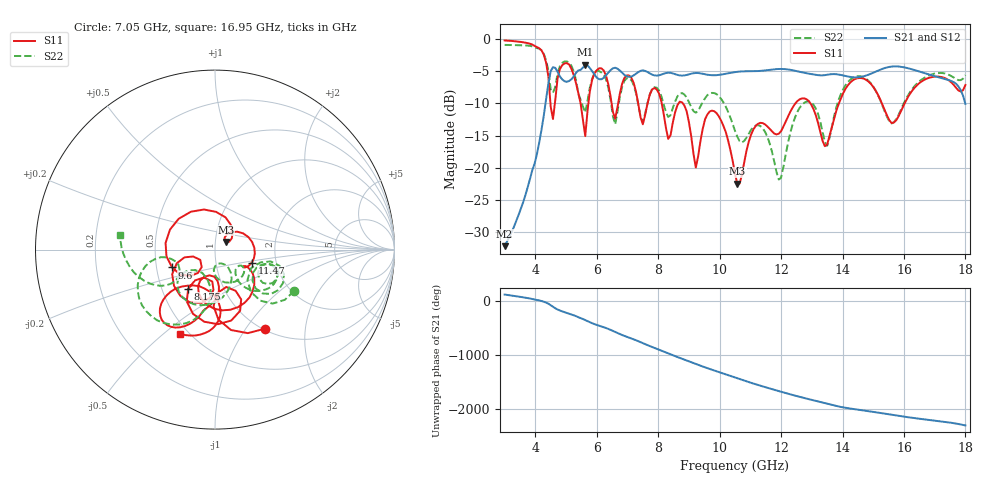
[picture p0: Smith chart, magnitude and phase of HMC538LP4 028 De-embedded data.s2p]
! Chelmsford, MA 01824
! http://www.hittite.com
! Tel: 978-250-3343
! Fax: 978-250-3373
! Device  :  HMC538LP4
! Description:  600 Analog Phase Shifter
! Frequency  :  6.0 GHz - 15.0 GHz
! Package  :  LP4  - 4x4 mm Quad Flatpack No-Lead (QFN) Plastic Package: 24 pin
! Ports  :  2 RF, 1 DC
!  Pin  3  = Rfin  = Port 1
!  Pin  16  = Rfout = Port 2
!  pin  21  = vCTL
! Voltages:  VCTL  = 0 to 5.0 Volts
! Currents :  Vb(V)  Vd(V)  Ib(mA)  Id(mA)
!  0.00  2.80  0.000000	0.471374
! Data:  The device was measured on evaluation board 111296-1.
!  Data was collected using a calibrated network analyzer.
!  The evaluation circuit board was modeled and simulated.This was use
!  to removed the evaluation board circuit from the measured data.
!  The reference plane is the center of the package pin.
! Misc:  Lot #
!Date Measured:  03 - 11 -2009
! Date:  03 - 17 -2009
! Note:
!  Hittite Microwave supplies this data as a sample of measured data at the
!  package pin for this package product.  Your particular data for this product
!  may vary.
!  Data was taken at 25 degrees C.
!  Hittite Microwave reserves the right to change this data at anytime.
# MHz S MA R 50
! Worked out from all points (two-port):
!   201 points, 3 GHz to 18 GHz, reference 50 ohm
!   highest |S21| = -4.00 dB at 5.625 GHz (marker M1); lowest = -32.2 dB at 3 GHz (marker M2)
!   |S21| within 3 dB of the highest: 4.422 GHz to 17.71 GHz (13.28 GHz wide, 120 % of centre)
!   lowest |S11| = -22.5 dB at 10.57 GHz (marker M3), VSWR 1.16, Z = 56.3 + j4.89 ohm
!   |S11| at or under -10 dB: 8.8 GHz to 12.47 GHz (3.668 GHz wide, 34.5 % of centre); 12.95 GHz to 13.88 GHz (929 MHz wide, 6.92 % of centre); 15.28 GHz to 16.02 GHz (743.1 MHz wide, 4.75 % of centre)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
!   |S22| runs from -21.8 to -0.9 dB; largest |S21 - S12| = 0.0022
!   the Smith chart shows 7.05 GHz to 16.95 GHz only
!   S11 on the Smith chart (normalised r, x): 7.05 GHz: 1.02, -1.23; 8.175 GHz: 0.68, -0.32; 9.6 GHz: 0.60, -0.13; 11.47 GHz: 1.49, -0.23; 16.95 GHz: 0.45, -0.57
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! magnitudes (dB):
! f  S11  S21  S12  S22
! 3 GHz  -0.2  -32.2  -32.2  -0.9
! 4.2 GHz  -1.8  -14.1  -14.1  -1.8
! 4.5 GHz  -10.5  -5.0  -5.0  -7.8
! 5.025 GHz  -3.7  -6.7  -6.7  -3.5
! 5.55 GHz  -12.6  -4.4  -4.4  -10.5
! 5.625 GHz  -15.1  -4.0  -4.0  -11.4
! 5.925 GHz  -5.3  -5.5  -5.5  -5.3
! 6.6 GHz  -12.4  -4.5  -4.5  -13.3
! 7.05 GHz  -5.7  -5.9  -5.9  -6.1
! 8.025 GHz  -8.4  -5.6  -5.6  -8.0
! 8.175 GHz  -11.5  -5.4  -5.4  -10.1
! 8.85 GHz  -10.3  -5.7  -5.7  -8.6
! 9.225 GHz  -20.0  -5.3  -5.3  -11.5
! 9.6 GHz  -11.7  -5.5  -5.6  -8.7
! 10.5 GHz  -21.0  -5.1  -5.1  -14.3
! 10.57 GHz  -22.5  -5.1  -5.1  -15.2
! 11.47 GHz  -13.3  -4.9  -4.9  -14.4
! 11.93 GHz  -14.7  -4.7  -4.7  -21.8
! 13.05 GHz  -10.8  -5.5  -5.5  -10.2
! 15.53 GHz  -12.6  -4.3  -4.3  -12.8
! 16.95 GHz  -5.9  -5.7  -5.7  -5.4
! 18 GHz  -7.2  -10.1  -10.1  -5.6
